(* SV subscriber ASDU *)
{attribute 'analysis' := '-33'}
{attribute 'no_assign'}
{attribute 'no_explicit_call' := 'Direct call not allowed for type FB_SVRXASDU_IED_MUnn_LLN0_MSVCB01'}
FUNCTION_BLOCK FB_SVRXASDU_IED_MUnn_LLN0_MSVCB01 EXTENDS FB_GseSvAsduClass
VAR_OUTPUT
	Values: ST_SVDATA_IED_MUnn_LLN0_PhsMeas1; (* SV dataset values buffer in IEC 61850 network transfer format (big endian) *)
END_VAR
VAR
	bAdd: BOOL := THIS^.AddValuesToContainer(pValues:=ADR(Values), cbValues:=SIZEOF(Values)); (* Adds SV dataset values buffer to the ASDU *)
END_VAR

END_FUNCTION_BLOCK
